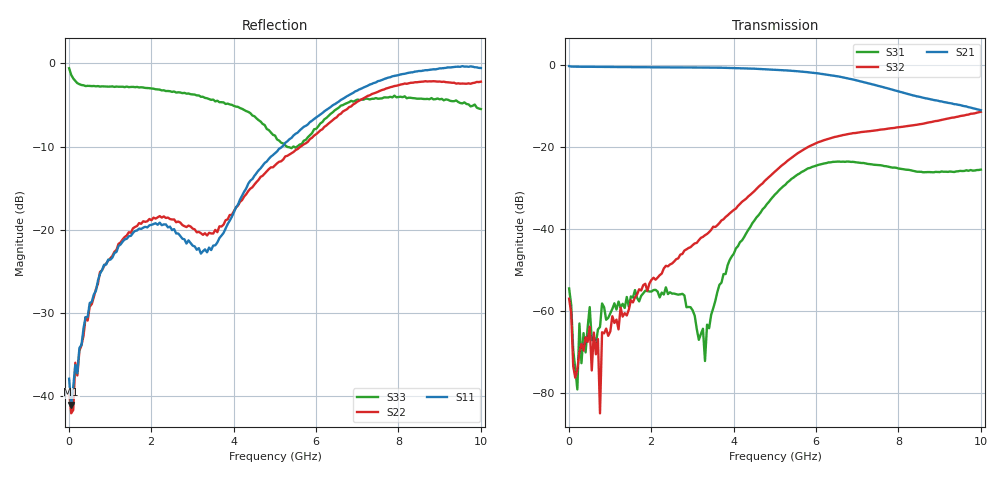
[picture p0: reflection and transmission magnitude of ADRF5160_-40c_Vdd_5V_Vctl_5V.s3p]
! Device:  ADRF5160
! Description: Silicon SPDT Switch
! Frequency:  0.7 -  4 GHz
! Ports:
!	RFc	= Port 1
!	RF1	= Port 2
!  RF2  = Port 3
! Vdd:  5 Volt
! Control:  5 Volt
! Data:  Data was collected using a calibrated 4 port network analyzer and de-embedded using Agilent's AFR De-Embedding.
! Note:  Analog Devices supplies this data as a sample of measured data
!  for this product.  Your particular data for this product may vary.
!  Data was taken at -40 degrees C.
!S3P File: Measurements: <S11,S12,S13>,
!<S21,S22,S23>,
!<S31,S32,S33>:
# Hz S  dB  R 50
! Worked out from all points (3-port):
!   201 points, 10 MHz to 10 GHz, reference 50 ohm
!   strongest paths, dB at 10 MHz, 2.507 GHz, 5.005 GHz, 7.503 GHz, 10 GHz:
!     S21: -0.4, -0.7, -1.2, -5.2, -11.1
!     S32: -57.1, -48.5, -26.1, -16.0, -11.5
!     S31: -54.6, -55.8, -31.7, -24.5, -25.6
!   lowest |S11| = -41.0 dB at 59.95 MHz (marker M1), VSWR 1.02, Z = 50.3 - j0.827 ohm
!   |S11| at or under -10 dB: start of sweep to 5.18 GHz
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1e7  -37.90 -27.7  -0.39 -0.1  -51.27 -24.5
     -0.37 -0.6  -39.33 -55.7  -65.57 -122.2
     -54.56 7.9  -57.07 9.7  -0.59 -8.6
5.995e7  -41.02 -67.5  -0.49 -1.8  -66.25 178.1
         -0.47 -1.7  -42.06 -63.1  -61.53 -90.2
         -58.52 99.3  -60.47 91.7  -1.38 -45.3
2.098e8  -37.24 -79.8  -0.50 -5.7  -69.80 -78.8
         -0.51 -5.7  -37.51 -86.1  -88.12 -145.6
         -79.20 -35.3  -74.38 -14.9  -2.38 -110.3
2.5975e8  -34.19 -84.8  -0.51 -6.9  -71.55 -81.7
          -0.51 -6.9  -34.53 -101.0  -67.84 174.0
          -63.12 17.9  -70.00 84.5  -2.50 -122.3
7.5925e8  -25.28 -101.5  -0.54 -20.0  -61.18 48.6
          -0.55 -20.0  -25.08 -118.7  -71.97 -84.7
          -63.95 74.9  -85.02 -140.1  -2.79 -172.0
8.092e8  -24.83 -104.5  -0.54 -21.3  -62.03 74.5
         -0.56 -21.3  -24.87 -118.8  -74.93 -104.0
         -58.23 89.6  -65.26 -98.3  -2.76 -174.8
2.35765e9  -19.36 -154.1  -0.66 -61.8  -54.93 64.6
           -0.67 -61.7  -18.58 -150.1  -49.27 -170.8
           -54.29 57.6  -49.05 -174.3  -3.33 140.7
3.3067e9  -22.35 136.1  -0.70 -87.6  -66.89 136.3
          -0.72 -87.6  -20.42 -141.5  -41.93 176.7
          -72.26 66.1  -41.60 176.9  -4.15 114.8
5.005e9  -10.80 16.6  -1.22 -138.1  -31.79 135.2
         -1.23 -138.0  -12.26 -121.7  -26.09 135.1
         -31.66 134.7  -26.06 135.1  -8.67 77.0
1e10  -0.56 -74.8  -11.08 88.9  -25.61 -83.0
      -11.11 89.1  -2.20 70.6  -11.50 -80.4
      -25.60 -83.2  -11.50 -80.4  -5.49 -15.2
